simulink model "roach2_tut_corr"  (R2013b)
settings: Solver=VariableStepDiscrete  SolverMode=SingleTasking  StartTime=0.0  StopTime=100  RelTol=1e-3
undefined symbols (not defined in the file): add_latency, addr_width, Bit, bitfield, BitWidth, bram_latency, burst_size, casper_library_scopes, conv_latency, data_width, DelayLen, fan_latency, FFTSize, FFTStage, getfield, increment, led, Location, Lower, mult_latency, mux_latency, n_bits, n_bits_data, n_inputs, n_streams, n_taps, neg_latency, negate_latency, nsamples, pfb_size, pulse_len, reset_period, ROACH, ROACH2, snapshot, sx475t, sync_period, sync_period_bits, Upper, UseCounter, Width
libraries: xbsIndex_r4 x24444, casper_library_misc x73, xbsReplacements_r4 x34, casper_library_delays x14, xps_library x7
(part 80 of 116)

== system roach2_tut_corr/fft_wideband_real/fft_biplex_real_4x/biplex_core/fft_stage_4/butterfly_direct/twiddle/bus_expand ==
  bus_in : Inport
  reinterpret1 : xbsIndex_r4/Reinterpret  force_arith_type=on  arith_type=Unsigned  force_bin_pt=on  bin_pt=0  block_type=reinterpret
  reinterpret2 : xbsIndex_r4/Reinterpret  force_arith_type=on  arith_type=Unsigned  force_bin_pt=on  bin_pt=0  block_type=reinterpret
  slice1 : xbsIndex_r4/Slice  nbits=145  boolean_output=off  mode=Upper Bit Location + Width  bit1=-144  base1=MSB of Input  bit0=0  base0=LSB of Input  dbl_ovrd=off  block_type=slice
  slice2 : xbsIndex_r4/Slice  nbits=144  boolean_output=off  mode=Upper Bit Location + Width  bit1=0  base1=MSB of Input  bit0=0  base0=LSB of Input  dbl_ovrd=off  block_type=slice
  msb_out2 : Outport
  lsb_out1 : Outport  Port=2
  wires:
  bus_in/1 -> slice2/1, slice1/1
  slice2/1 -> reinterpret2/1
  reinterpret2/1 -> msb_out2/1
  slice1/1 -> reinterpret1/1
  reinterpret1/1 -> lsb_out1/1

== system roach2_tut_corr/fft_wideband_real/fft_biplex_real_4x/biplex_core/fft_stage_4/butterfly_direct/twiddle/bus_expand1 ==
  bus_in : Inport
  reinterpret1 : xbsIndex_r4/Reinterpret  force_arith_type=on  arith_type=Unsigned  force_bin_pt=on  bin_pt=0  block_type=reinterpret
  slice1 : xbsIndex_r4/Slice  nbits=144  boolean_output=off  mode=Upper Bit Location + Width  bit1=-1  base1=MSB of Input  bit0=0  base0=LSB of Input  dbl_ovrd=off  block_type=slice
  slice2 : xbsIndex_r4/Slice  nbits=1  boolean_output=on  mode=Upper Bit Location + Width  bit1=0  base1=MSB of Input  bit0=0  base0=LSB of Input  dbl_ovrd=off  block_type=slice
  msb_out2 : Outport
  lsb_out1 : Outport  Port=2
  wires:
  bus_in/1 -> slice2/1, slice1/1
  slice2/1 -> msb_out2/1
  slice1/1 -> reinterpret1/1
  reinterpret1/1 -> lsb_out1/1

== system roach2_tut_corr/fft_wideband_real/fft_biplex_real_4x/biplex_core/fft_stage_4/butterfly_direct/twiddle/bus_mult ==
  a : Inport
  b : Inport  Port=2
  misci : Inport  Port=3
  a*b_bussify : Subsystem  AncestorBlock=casper_library_flow_control/bus_create
  a_debus : Subsystem  AncestorBlock=casper_library_flow_control/bus_expand
  b_debus : Subsystem  AncestorBlock=casper_library_flow_control/bus_expand
  dmisc : xbsIndex_r4/Delay  rst=off  infoeditControl=Selection of Reset will increase slice count due to use of real FFs and instead of SRLs  en=off  latency=mult_latency+add_latency+conv_latency+fan_latency  dbl_ovrd=off  reg_retiming=on  block_type=delay
  mult1 : Subsystem  AncestorBlock=casper_library_multipliers/cmult
  mult2 : Subsystem  AncestorBlock=casper_library_multipliers/cmult
  mult3 : Subsystem  AncestorBlock=casper_library_multipliers/cmult
  mult4 : Subsystem  AncestorBlock=casper_library_multipliers/cmult
  repa : Subsystem  AncestorBlock=casper_library_bus/bus_replicate
  repb : Subsystem  AncestorBlock=casper_library_bus/bus_replicate
  a*b : Outport
  misco : Outport  Port=2
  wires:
  a/1 -> repa/1(in)
  b/1 -> repb/1(in)
  repa/1(out) -> a_debus/1(bus_in)
  repb/1(out) -> b_debus/1(bus_in)
  a_debus/1(msb_lsb_out1) -> mult1/1(a), mult2/1(a), mult3/1(a), mult4/1(a)
  b_debus/1(msb_out4) -> mult1/2(b)
  b_debus/2(out3) -> mult2/2(b)
  b_debus/3(out2) -> mult3/2(b)
  b_debus/4(lsb_out1) -> mult4/2(b)
  misci/1 -> dmisc/1
  mult1/1(ab) -> a*b_bussify/1(in1)
  mult2/1(ab) -> a*b_bussify/2(in2)
  mult3/1(ab) -> a*b_bussify/3(in3)
  mult4/1(ab) -> a*b_bussify/4(in4)
  a*b_bussify/1(bus_out) -> a*b/1
  dmisc/1 -> misco/1

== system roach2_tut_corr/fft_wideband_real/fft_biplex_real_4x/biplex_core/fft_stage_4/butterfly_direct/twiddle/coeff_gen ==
  rst : Inport
  misci : Inport  Port=2
  Counter : xbsIndex_r4/Counter  cnt_type=Free Running  cnt_to=Inf  operation=Up  start_count=0  cnt_by_val=1  arith_type=Unsigned  n_bits=8  bin_pt=0  load_pin=off  rst=on  en=off  explicit_period=on  period=1  dbl_ovrd=off  use_behavioral_HDL=on  implementation=Fabric  block_type=counter
  Slice : xbsIndex_r4/Slice  nbits=3  boolean_output=off  mode=Upper Bit Location + Width  bit1=0  base1=MSB of Input  bit0=0  base0=LSB of Input  dbl_ovrd=off  block_type=slice
  bit_reverse : Subsystem  AncestorBlock=casper_library_misc/bit_reverse
  cosin : Subsystem  Tag=casper:cosin  AncestorBlock=casper_library_downconverter/cosin
  ri_to_c : casper_library_misc/ri_to_c
  w : Outport
  misco : Outport  Port=2
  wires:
  ri_to_c/1 -> w/1
  rst/1 -> Counter/1
  Counter/1 -> Slice/1
  Slice/1 -> bit_reverse/1(in)
  bit_reverse/1(out) -> cosin/1(theta)
  cosin/1(cos) -> ri_to_c/1
  cosin/2(-sin) -> ri_to_c/2
  misci/1 -> cosin/2(misci)
  cosin/3(misco) -> misco/1

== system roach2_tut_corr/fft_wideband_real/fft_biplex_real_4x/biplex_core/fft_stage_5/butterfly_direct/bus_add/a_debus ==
  bus_in : Inport
  reinterpret{1..8} (8 alike) : xbsIndex_r4/Reinterpret  force_arith_type=on  arith_type="Signed  (2's comp)"  force_bin_pt=on  bin_pt=17  block_type=reinterpret
  slice1 : xbsIndex_r4/Slice  nbits=18  boolean_output=off  mode=Upper Bit Location + Width  bit1=-126  base1=MSB of Input  bit0=0  base0=LSB of Input  dbl_ovrd=off  block_type=slice
  slice2 : xbsIndex_r4/Slice  nbits=18  boolean_output=off  mode=Upper Bit Location + Width  bit1=-108  base1=MSB of Input  bit0=0  base0=LSB of Input  dbl_ovrd=off  block_type=slice
  slice3 : xbsIndex_r4/Slice  nbits=18  boolean_output=off  mode=Upper Bit Location + Width  bit1=-90  base1=MSB of Input  bit0=0  base0=LSB of Input  dbl_ovrd=off  block_type=slice
  slice4 : xbsIndex_r4/Slice  nbits=18  boolean_output=off  mode=Upper Bit Location + Width  bit1=-72  base1=MSB of Input  bit0=0  base0=LSB of Input  dbl_ovrd=off  block_type=slice
  slice5 : xbsIndex_r4/Slice  nbits=18  boolean_output=off  mode=Upper Bit Location + Width  bit1=-54  base1=MSB of Input  bit0=0  base0=LSB of Input  dbl_ovrd=off  block_type=slice
  slice6 : xbsIndex_r4/Slice  nbits=18  boolean_output=off  mode=Upper Bit Location + Width  bit1=-36  base1=MSB of Input  bit0=0  base0=LSB of Input  dbl_ovrd=off  block_type=slice
  slice7 : xbsIndex_r4/Slice  nbits=18  boolean_output=off  mode=Upper Bit Location + Width  bit1=-18  base1=MSB of Input  bit0=0  base0=LSB of Input  dbl_ovrd=off  block_type=slice
  slice8 : xbsIndex_r4/Slice  nbits=18  boolean_output=off  mode=Upper Bit Location + Width  bit1=0  base1=MSB of Input  bit0=0  base0=LSB of Input  dbl_ovrd=off  block_type=slice
  msb_out8 : Outport
  out7 : Outport  Port=2
  out6 : Outport  Port=3
  out5 : Outport  Port=4
  out4 : Outport  Port=5
  out3 : Outport  Port=6
  out2 : Outport  Port=7
  lsb_out1 : Outport  Port=8
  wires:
  bus_in/1 -> slice8/1, slice7/1, slice6/1, slice5/1, slice4/1, slice3/1, slice2/1, slice1/1
  slice8/1 -> reinterpret8/1
  reinterpret8/1 -> msb_out8/1
  slice7/1 -> reinterpret7/1
  reinterpret7/1 -> out7/1
  slice6/1 -> reinterpret6/1
  reinterpret6/1 -> out6/1
  slice5/1 -> reinterpret5/1
  reinterpret5/1 -> out5/1
  slice4/1 -> reinterpret4/1
  reinterpret4/1 -> out4/1
  slice3/1 -> reinterpret3/1
  reinterpret3/1 -> out3/1
  slice2/1 -> reinterpret2/1
  reinterpret2/1 -> out2/1
  slice1/1 -> reinterpret1/1
  reinterpret1/1 -> lsb_out1/1

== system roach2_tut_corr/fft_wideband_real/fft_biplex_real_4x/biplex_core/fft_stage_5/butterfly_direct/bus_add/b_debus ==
  bus_in : Inport
  reinterpret{1..8} (8 alike) : xbsIndex_r4/Reinterpret  force_arith_type=on  arith_type="Signed  (2's comp)"  force_bin_pt=on  bin_pt=17  block_type=reinterpret
  slice1 : xbsIndex_r4/Slice  nbits=19  boolean_output=off  mode=Upper Bit Location + Width  bit1=-133  base1=MSB of Input  bit0=0  base0=LSB of Input  dbl_ovrd=off  block_type=slice
  slice2 : xbsIndex_r4/Slice  nbits=19  boolean_output=off  mode=Upper Bit Location + Width  bit1=-114  base1=MSB of Input  bit0=0  base0=LSB of Input  dbl_ovrd=off  block_type=slice
  slice3 : xbsIndex_r4/Slice  nbits=19  boolean_output=off  mode=Upper Bit Location + Width  bit1=-95  base1=MSB of Input  bit0=0  base0=LSB of Input  dbl_ovrd=off  block_type=slice
  slice4 : xbsIndex_r4/Slice  nbits=19  boolean_output=off  mode=Upper Bit Location + Width  bit1=-76  base1=MSB of Input  bit0=0  base0=LSB of Input  dbl_ovrd=off  block_type=slice
  slice5 : xbsIndex_r4/Slice  nbits=19  boolean_output=off  mode=Upper Bit Location + Width  bit1=-57  base1=MSB of Input  bit0=0  base0=LSB of Input  dbl_ovrd=off  block_type=slice
  slice6 : xbsIndex_r4/Slice  nbits=19  boolean_output=off  mode=Upper Bit Location + Width  bit1=-38  base1=MSB of Input  bit0=0  base0=LSB of Input  dbl_ovrd=off  block_type=slice
  slice7 : xbsIndex_r4/Slice  nbits=19  boolean_output=off  mode=Upper Bit Location + Width  bit1=-19  base1=MSB of Input  bit0=0  base0=LSB of Input  dbl_ovrd=off  block_type=slice
  slice8 : xbsIndex_r4/Slice  nbits=19  boolean_output=off  mode=Upper Bit Location + Width  bit1=0  base1=MSB of Input  bit0=0  base0=LSB of Input  dbl_ovrd=off  block_type=slice
  msb_out8 : Outport
  out7 : Outport  Port=2
  out6 : Outport  Port=3
  out5 : Outport  Port=4
  out4 : Outport  Port=5
  out3 : Outport  Port=6
  out2 : Outport  Port=7
  lsb_out1 : Outport  Port=8
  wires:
  bus_in/1 -> slice8/1, slice7/1, slice6/1, slice5/1, slice4/1, slice3/1, slice2/1, slice1/1
  slice8/1 -> reinterpret8/1
  reinterpret8/1 -> msb_out8/1
  slice7/1 -> reinterpret7/1
  reinterpret7/1 -> out7/1
  slice6/1 -> reinterpret6/1
  reinterpret6/1 -> out6/1
  slice5/1 -> reinterpret5/1
  reinterpret5/1 -> out5/1
  slice4/1 -> reinterpret4/1
  reinterpret4/1 -> out4/1
  slice3/1 -> reinterpret3/1
  reinterpret3/1 -> out3/1
  slice2/1 -> reinterpret2/1
  reinterpret2/1 -> out2/1
  slice1/1 -> reinterpret1/1
  reinterpret1/1 -> lsb_out1/1

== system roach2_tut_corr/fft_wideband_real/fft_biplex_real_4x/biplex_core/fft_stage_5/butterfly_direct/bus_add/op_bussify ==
  in1 : Inport
  in2 : Inport  Port=2
  in3 : Inport  Port=3
  in4 : Inport  Port=4
  in5 : Inport  Port=5
  in6 : Inport  Port=6
  in7 : Inport  Port=7
  in8 : Inport  Port=8
  concatenate : xbsIndex_r4/Concat  num_inputs=8  dbl_ovrd=off  block_type=concat
  reinterpret{1..8} (8 alike) : xbsIndex_r4/Reinterpret  force_arith_type=on  arith_type=Unsigned  force_bin_pt=on  bin_pt=0  block_type=reinterpret
  bus_out : Outport
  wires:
  concatenate/1 -> bus_out/1
  in1/1 -> reinterpret1/1
  reinterpret1/1 -> concatenate/1
  in2/1 -> reinterpret2/1
  reinterpret2/1 -> concatenate/2
  in3/1 -> reinterpret3/1
  reinterpret3/1 -> concatenate/3
  in4/1 -> reinterpret4/1
  reinterpret4/1 -> concatenate/4
  in5/1 -> reinterpret5/1
  reinterpret5/1 -> concatenate/5
  in6/1 -> reinterpret6/1
  reinterpret6/1 -> concatenate/6
  in7/1 -> reinterpret7/1
  reinterpret7/1 -> concatenate/7
  in8/1 -> reinterpret8/1
  reinterpret8/1 -> concatenate/8

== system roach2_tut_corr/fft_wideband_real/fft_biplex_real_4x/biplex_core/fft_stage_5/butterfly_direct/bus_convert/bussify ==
  in1 : Inport
  in2 : Inport  Port=2
  in3 : Inport  Port=3
  in4 : Inport  Port=4
  in5 : Inport  Port=5
  in6 : Inport  Port=6
  in7 : Inport  Port=7
  in8 : Inport  Port=8
  in9 : Inport  Port=9
  in10 : Inport  Port=10
  in11 : Inport  Port=11
  in12 : Inport  Port=12
  in13 : Inport  Port=13
  in14 : Inport  Port=14
  in15 : Inport  Port=15
  in16 : Inport  Port=16
  concatenate : xbsIndex_r4/Concat  num_inputs=16  dbl_ovrd=off  block_type=concat
  reinterpret{1..16} (16 alike) : xbsIndex_r4/Reinterpret  force_arith_type=on  arith_type=Unsigned  force_bin_pt=on  bin_pt=0  block_type=reinterpret
  bus_out : Outport
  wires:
  concatenate/1 -> bus_out/1
  in1/1 -> reinterpret1/1
  reinterpret1/1 -> concatenate/1
  in2/1 -> reinterpret2/1
  reinterpret2/1 -> concatenate/2
  in3/1 -> reinterpret3/1
  reinterpret3/1 -> concatenate/3
  in4/1 -> reinterpret4/1
  reinterpret4/1 -> concatenate/4
  in5/1 -> reinterpret5/1
  reinterpret5/1 -> concatenate/5
  in6/1 -> reinterpret6/1
  reinterpret6/1 -> concatenate/6
  in7/1 -> reinterpret7/1
  reinterpret7/1 -> concatenate/7
  in8/1 -> reinterpret8/1
  reinterpret8/1 -> concatenate/8
  in9/1 -> reinterpret9/1
  reinterpret9/1 -> concatenate/9
  in10/1 -> reinterpret10/1
  reinterpret10/1 -> concatenate/10
  in11/1 -> reinterpret11/1
  reinterpret11/1 -> concatenate/11
  in12/1 -> reinterpret12/1
  reinterpret12/1 -> concatenate/12
  in13/1 -> reinterpret13/1
  reinterpret13/1 -> concatenate/13
  in14/1 -> reinterpret14/1
  reinterpret14/1 -> concatenate/14
  in15/1 -> reinterpret15/1
  reinterpret15/1 -> concatenate/15
  in16/1 -> reinterpret16/1
  reinterpret16/1 -> concatenate/16

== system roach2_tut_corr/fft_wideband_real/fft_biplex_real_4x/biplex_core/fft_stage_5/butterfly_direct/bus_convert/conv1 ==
  din : Inport
  all_0s : xbsIndex_r4/Logical  logical_function=NAND  inputs=3  en=off  latency=1  precision=Full  arith_type=Unsigned  n_bits=16  bin_pt=0  align_bp=on  dbl_ovrd=off  block_type=logical
  all_1s : xbsIndex_r4/Logical  logical_function=NAND  inputs=3  en=off  latency=1  precision=Full  arith_type=Unsigned  n_bits=16  bin_pt=0  align_bp=on  dbl_ovrd=off  block_type=logical
  and : xbsIndex_r4/Logical  logical_function=AND  inputs=2  en=off  latency=0  precision=Full  arith_type=Unsigned  n_bits=16  bin_pt=0  align_bp=on  dbl_ovrd=off  block_type=logical
  convert : Subsystem  AncestorBlock=casper_library_misc/convert
  invert1 : xbsIndex_r4/Inverter  en=off  latency=0  dbl_ovrd=off  block_type=inv
  invert2 : xbsIndex_r4/Inverter  en=off  latency=0  dbl_ovrd=off  block_type=inv
  invert3 : xbsIndex_r4/Inverter  en=off  latency=0  dbl_ovrd=off  block_type=inv
  slice1 : xbsIndex_r4/Slice  nbits=1  boolean_output=on  mode=Upper Bit Location + Width  bit1=0  base1=MSB of Input  bit0=0  base0=LSB of Input  dbl_ovrd=off  block_type=slice
  slice2 : xbsIndex_r4/Slice  nbits=1  boolean_output=on  mode=Upper Bit Location + Width  bit1=-1  base1=MSB of Input  bit0=0  base0=LSB of Input  dbl_ovrd=off  block_type=slice
  slice3 : xbsIndex_r4/Slice  nbits=1  boolean_output=on  mode=Upper Bit Location + Width  bit1=-2  base1=MSB of Input  bit0=0  base0=LSB of Input  dbl_ovrd=off  block_type=slice
  dout : Outport
  of : Outport  Port=2
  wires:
  din/1 -> convert/1(in), slice1/1, slice2/1, slice3/1
  convert/1(out) -> dout/1
  slice1/1 -> all_1s/1, invert1/1
  invert1/1 -> all_0s/1
  slice2/1 -> all_1s/2, invert2/1
  invert2/1 -> all_0s/2
  slice3/1 -> all_1s/3, invert3/1
  invert3/1 -> all_0s/3
  all_0s/1 -> and/1
  all_1s/1 -> and/2
  and/1 -> of/1

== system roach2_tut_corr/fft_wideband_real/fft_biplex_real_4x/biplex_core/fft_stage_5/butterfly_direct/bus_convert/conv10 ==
  din : Inport
  all_0s : xbsIndex_r4/Logical  logical_function=NAND  inputs=3  en=off  latency=1  precision=Full  arith_type=Unsigned  n_bits=16  bin_pt=0  align_bp=on  dbl_ovrd=off  block_type=logical
  all_1s : xbsIndex_r4/Logical  logical_function=NAND  inputs=3  en=off  latency=1  precision=Full  arith_type=Unsigned  n_bits=16  bin_pt=0  align_bp=on  dbl_ovrd=off  block_type=logical
  and : xbsIndex_r4/Logical  logical_function=AND  inputs=2  en=off  latency=0  precision=Full  arith_type=Unsigned  n_bits=16  bin_pt=0  align_bp=on  dbl_ovrd=off  block_type=logical
  convert : Subsystem  AncestorBlock=casper_library_misc/convert
  invert1 : xbsIndex_r4/Inverter  en=off  latency=0  dbl_ovrd=off  block_type=inv
  invert2 : xbsIndex_r4/Inverter  en=off  latency=0  dbl_ovrd=off  block_type=inv
  invert3 : xbsIndex_r4/Inverter  en=off  latency=0  dbl_ovrd=off  block_type=inv
  slice1 : xbsIndex_r4/Slice  nbits=1  boolean_output=on  mode=Upper Bit Location + Width  bit1=0  base1=MSB of Input  bit0=0  base0=LSB of Input  dbl_ovrd=off  block_type=slice
  slice2 : xbsIndex_r4/Slice  nbits=1  boolean_output=on  mode=Upper Bit Location + Width  bit1=-1  base1=MSB of Input  bit0=0  base0=LSB of Input  dbl_ovrd=off  block_type=slice
  slice3 : xbsIndex_r4/Slice  nbits=1  boolean_output=on  mode=Upper Bit Location + Width  bit1=-2  base1=MSB of Input  bit0=0  base0=LSB of Input  dbl_ovrd=off  block_type=slice
  dout : Outport
  of : Outport  Port=2
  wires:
  din/1 -> convert/1(in), slice1/1, slice2/1, slice3/1
  convert/1(out) -> dout/1
  slice1/1 -> all_1s/1, invert1/1
  invert1/1 -> all_0s/1
  slice2/1 -> all_1s/2, invert2/1
  invert2/1 -> all_0s/2
  slice3/1 -> all_1s/3, invert3/1
  invert3/1 -> all_0s/3
  all_0s/1 -> and/1
  all_1s/1 -> and/2
  and/1 -> of/1

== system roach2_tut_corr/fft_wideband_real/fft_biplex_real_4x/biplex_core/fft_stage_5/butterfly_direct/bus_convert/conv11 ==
  din : Inport
  all_0s : xbsIndex_r4/Logical  logical_function=NAND  inputs=3  en=off  latency=1  precision=Full  arith_type=Unsigned  n_bits=16  bin_pt=0  align_bp=on  dbl_ovrd=off  block_type=logical
  all_1s : xbsIndex_r4/Logical  logical_function=NAND  inputs=3  en=off  latency=1  precision=Full  arith_type=Unsigned  n_bits=16  bin_pt=0  align_bp=on  dbl_ovrd=off  block_type=logical
  and : xbsIndex_r4/Logical  logical_function=AND  inputs=2  en=off  latency=0  precision=Full  arith_type=Unsigned  n_bits=16  bin_pt=0  align_bp=on  dbl_ovrd=off  block_type=logical
  convert : Subsystem  AncestorBlock=casper_library_misc/convert
  invert1 : xbsIndex_r4/Inverter  en=off  latency=0  dbl_ovrd=off  block_type=inv
  invert2 : xbsIndex_r4/Inverter  en=off  latency=0  dbl_ovrd=off  block_type=inv
  invert3 : xbsIndex_r4/Inverter  en=off  latency=0  dbl_ovrd=off  block_type=inv
  slice1 : xbsIndex_r4/Slice  nbits=1  boolean_output=on  mode=Upper Bit Location + Width  bit1=0  base1=MSB of Input  bit0=0  base0=LSB of Input  dbl_ovrd=off  block_type=slice
  slice2 : xbsIndex_r4/Slice  nbits=1  boolean_output=on  mode=Upper Bit Location + Width  bit1=-1  base1=MSB of Input  bit0=0  base0=LSB of Input  dbl_ovrd=off  block_type=slice
  slice3 : xbsIndex_r4/Slice  nbits=1  boolean_output=on  mode=Upper Bit Location + Width  bit1=-2  base1=MSB of Input  bit0=0  base0=LSB of Input  dbl_ovrd=off  block_type=slice
  dout : Outport
  of : Outport  Port=2
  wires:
  din/1 -> convert/1(in), slice1/1, slice2/1, slice3/1
  convert/1(out) -> dout/1
  slice1/1 -> all_1s/1, invert1/1
  invert1/1 -> all_0s/1
  slice2/1 -> all_1s/2, invert2/1
  invert2/1 -> all_0s/2
  slice3/1 -> all_1s/3, invert3/1
  invert3/1 -> all_0s/3
  all_0s/1 -> and/1
  all_1s/1 -> and/2
  and/1 -> of/1

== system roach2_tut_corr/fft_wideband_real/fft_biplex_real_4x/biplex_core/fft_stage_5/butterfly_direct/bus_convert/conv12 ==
  din : Inport
  all_0s : xbsIndex_r4/Logical  logical_function=NAND  inputs=3  en=off  latency=1  precision=Full  arith_type=Unsigned  n_bits=16  bin_pt=0  align_bp=on  dbl_ovrd=off  block_type=logical
  all_1s : xbsIndex_r4/Logical  logical_function=NAND  inputs=3  en=off  latency=1  precision=Full  arith_type=Unsigned  n_bits=16  bin_pt=0  align_bp=on  dbl_ovrd=off  block_type=logical
  and : xbsIndex_r4/Logical  logical_function=AND  inputs=2  en=off  latency=0  precision=Full  arith_type=Unsigned  n_bits=16  bin_pt=0  align_bp=on  dbl_ovrd=off  block_type=logical
  convert : Subsystem  AncestorBlock=casper_library_misc/convert
  invert1 : xbsIndex_r4/Inverter  en=off  latency=0  dbl_ovrd=off  block_type=inv
  invert2 : xbsIndex_r4/Inverter  en=off  latency=0  dbl_ovrd=off  block_type=inv
  invert3 : xbsIndex_r4/Inverter  en=off  latency=0  dbl_ovrd=off  block_type=inv
  slice1 : xbsIndex_r4/Slice  nbits=1  boolean_output=on  mode=Upper Bit Location + Width  bit1=0  base1=MSB of Input  bit0=0  base0=LSB of Input  dbl_ovrd=off  block_type=slice
  slice2 : xbsIndex_r4/Slice  nbits=1  boolean_output=on  mode=Upper Bit Location + Width  bit1=-1  base1=MSB of Input  bit0=0  base0=LSB of Input  dbl_ovrd=off  block_type=slice
  slice3 : xbsIndex_r4/Slice  nbits=1  boolean_output=on  mode=Upper Bit Location + Width  bit1=-2  base1=MSB of Input  bit0=0  base0=LSB of Input  dbl_ovrd=off  block_type=slice
  dout : Outport
  of : Outport  Port=2
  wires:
  din/1 -> convert/1(in), slice1/1, slice2/1, slice3/1
  convert/1(out) -> dout/1
  slice1/1 -> all_1s/1, invert1/1
  invert1/1 -> all_0s/1
  slice2/1 -> all_1s/2, invert2/1
  invert2/1 -> all_0s/2
  slice3/1 -> all_1s/3, invert3/1
  invert3/1 -> all_0s/3
  all_0s/1 -> and/1
  all_1s/1 -> and/2
  and/1 -> of/1

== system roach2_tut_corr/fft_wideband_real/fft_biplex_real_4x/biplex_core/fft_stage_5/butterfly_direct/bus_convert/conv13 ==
  din : Inport
  all_0s : xbsIndex_r4/Logical  logical_function=NAND  inputs=3  en=off  latency=1  precision=Full  arith_type=Unsigned  n_bits=16  bin_pt=0  align_bp=on  dbl_ovrd=off  block_type=logical
  all_1s : xbsIndex_r4/Logical  logical_function=NAND  inputs=3  en=off  latency=1  precision=Full  arith_type=Unsigned  n_bits=16  bin_pt=0  align_bp=on  dbl_ovrd=off  block_type=logical
  and : xbsIndex_r4/Logical  logical_function=AND  inputs=2  en=off  latency=0  precision=Full  arith_type=Unsigned  n_bits=16  bin_pt=0  align_bp=on  dbl_ovrd=off  block_type=logical
  convert : Subsystem  AncestorBlock=casper_library_misc/convert
  invert1 : xbsIndex_r4/Inverter  en=off  latency=0  dbl_ovrd=off  block_type=inv
  invert2 : xbsIndex_r4/Inverter  en=off  latency=0  dbl_ovrd=off  block_type=inv
  invert3 : xbsIndex_r4/Inverter  en=off  latency=0  dbl_ovrd=off  block_type=inv
  slice1 : xbsIndex_r4/Slice  nbits=1  boolean_output=on  mode=Upper Bit Location + Width  bit1=0  base1=MSB of Input  bit0=0  base0=LSB of Input  dbl_ovrd=off  block_type=slice
  slice2 : xbsIndex_r4/Slice  nbits=1  boolean_output=on  mode=Upper Bit Location + Width  bit1=-1  base1=MSB of Input  bit0=0  base0=LSB of Input  dbl_ovrd=off  block_type=slice
  slice3 : xbsIndex_r4/Slice  nbits=1  boolean_output=on  mode=Upper Bit Location + Width  bit1=-2  base1=MSB of Input  bit0=0  base0=LSB of Input  dbl_ovrd=off  block_type=slice
  dout : Outport
  of : Outport  Port=2
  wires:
  din/1 -> convert/1(in), slice1/1, slice2/1, slice3/1
  convert/1(out) -> dout/1
  slice1/1 -> all_1s/1, invert1/1
  invert1/1 -> all_0s/1
  slice2/1 -> all_1s/2, invert2/1
  invert2/1 -> all_0s/2
  slice3/1 -> all_1s/3, invert3/1
  invert3/1 -> all_0s/3
  all_0s/1 -> and/1
  all_1s/1 -> and/2
  and/1 -> of/1

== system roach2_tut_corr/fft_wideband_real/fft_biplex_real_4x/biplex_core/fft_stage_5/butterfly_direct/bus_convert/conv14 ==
  din : Inport
  all_0s : xbsIndex_r4/Logical  logical_function=NAND  inputs=3  en=off  latency=1  precision=Full  arith_type=Unsigned  n_bits=16  bin_pt=0  align_bp=on  dbl_ovrd=off  block_type=logical
  all_1s : xbsIndex_r4/Logical  logical_function=NAND  inputs=3  en=off  latency=1  precision=Full  arith_type=Unsigned  n_bits=16  bin_pt=0  align_bp=on  dbl_ovrd=off  block_type=logical
  and : xbsIndex_r4/Logical  logical_function=AND  inputs=2  en=off  latency=0  precision=Full  arith_type=Unsigned  n_bits=16  bin_pt=0  align_bp=on  dbl_ovrd=off  block_type=logical
  convert : Subsystem  AncestorBlock=casper_library_misc/convert
  invert1 : xbsIndex_r4/Inverter  en=off  latency=0  dbl_ovrd=off  block_type=inv
  invert2 : xbsIndex_r4/Inverter  en=off  latency=0  dbl_ovrd=off  block_type=inv
  invert3 : xbsIndex_r4/Inverter  en=off  latency=0  dbl_ovrd=off  block_type=inv
  slice1 : xbsIndex_r4/Slice  nbits=1  boolean_output=on  mode=Upper Bit Location + Width  bit1=0  base1=MSB of Input  bit0=0  base0=LSB of Input  dbl_ovrd=off  block_type=slice
  slice2 : xbsIndex_r4/Slice  nbits=1  boolean_output=on  mode=Upper Bit Location + Width  bit1=-1  base1=MSB of Input  bit0=0  base0=LSB of Input  dbl_ovrd=off  block_type=slice
  slice3 : xbsIndex_r4/Slice  nbits=1  boolean_output=on  mode=Upper Bit Location + Width  bit1=-2  base1=MSB of Input  bit0=0  base0=LSB of Input  dbl_ovrd=off  block_type=slice
  dout : Outport
  of : Outport  Port=2
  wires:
  din/1 -> convert/1(in), slice1/1, slice2/1, slice3/1
  convert/1(out) -> dout/1
  slice1/1 -> all_1s/1, invert1/1
  invert1/1 -> all_0s/1
  slice2/1 -> all_1s/2, invert2/1
  invert2/1 -> all_0s/2
  slice3/1 -> all_1s/3, invert3/1
  invert3/1 -> all_0s/3
  all_0s/1 -> and/1
  all_1s/1 -> and/2
  and/1 -> of/1

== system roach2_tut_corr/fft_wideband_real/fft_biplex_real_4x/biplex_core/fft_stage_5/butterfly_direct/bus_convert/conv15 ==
  din : Inport
  all_0s : xbsIndex_r4/Logical  logical_function=NAND  inputs=3  en=off  latency=1  precision=Full  arith_type=Unsigned  n_bits=16  bin_pt=0  align_bp=on  dbl_ovrd=off  block_type=logical
  all_1s : xbsIndex_r4/Logical  logical_function=NAND  inputs=3  en=off  latency=1  precision=Full  arith_type=Unsigned  n_bits=16  bin_pt=0  align_bp=on  dbl_ovrd=off  block_type=logical
  and : xbsIndex_r4/Logical  logical_function=AND  inputs=2  en=off  latency=0  precision=Full  arith_type=Unsigned  n_bits=16  bin_pt=0  align_bp=on  dbl_ovrd=off  block_type=logical
  convert : Subsystem  AncestorBlock=casper_library_misc/convert
  invert1 : xbsIndex_r4/Inverter  en=off  latency=0  dbl_ovrd=off  block_type=inv
  invert2 : xbsIndex_r4/Inverter  en=off  latency=0  dbl_ovrd=off  block_type=inv
  invert3 : xbsIndex_r4/Inverter  en=off  latency=0  dbl_ovrd=off  block_type=inv
  slice1 : xbsIndex_r4/Slice  nbits=1  boolean_output=on  mode=Upper Bit Location + Width  bit1=0  base1=MSB of Input  bit0=0  base0=LSB of Input  dbl_ovrd=off  block_type=slice
  slice2 : xbsIndex_r4/Slice  nbits=1  boolean_output=on  mode=Upper Bit Location + Width  bit1=-1  base1=MSB of Input  bit0=0  base0=LSB of Input  dbl_ovrd=off  block_type=slice
  slice3 : xbsIndex_r4/Slice  nbits=1  boolean_output=on  mode=Upper Bit Location + Width  bit1=-2  base1=MSB of Input  bit0=0  base0=LSB of Input  dbl_ovrd=off  block_type=slice
  dout : Outport
  of : Outport  Port=2
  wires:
  din/1 -> convert/1(in), slice1/1, slice2/1, slice3/1
  convert/1(out) -> dout/1
  slice1/1 -> all_1s/1, invert1/1
  invert1/1 -> all_0s/1
  slice2/1 -> all_1s/2, invert2/1
  invert2/1 -> all_0s/2
  slice3/1 -> all_1s/3, invert3/1
  invert3/1 -> all_0s/3
  all_0s/1 -> and/1
  all_1s/1 -> and/2
  and/1 -> of/1

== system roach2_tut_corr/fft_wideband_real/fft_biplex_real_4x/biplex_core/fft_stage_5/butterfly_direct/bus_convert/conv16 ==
  din : Inport
  all_0s : xbsIndex_r4/Logical  logical_function=NAND  inputs=3  en=off  latency=1  precision=Full  arith_type=Unsigned  n_bits=16  bin_pt=0  align_bp=on  dbl_ovrd=off  block_type=logical
  all_1s : xbsIndex_r4/Logical  logical_function=NAND  inputs=3  en=off  latency=1  precision=Full  arith_type=Unsigned  n_bits=16  bin_pt=0  align_bp=on  dbl_ovrd=off  block_type=logical
  and : xbsIndex_r4/Logical  logical_function=AND  inputs=2  en=off  latency=0  precision=Full  arith_type=Unsigned  n_bits=16  bin_pt=0  align_bp=on  dbl_ovrd=off  block_type=logical
  convert : Subsystem  AncestorBlock=casper_library_misc/convert
  invert1 : xbsIndex_r4/Inverter  en=off  latency=0  dbl_ovrd=off  block_type=inv
  invert2 : xbsIndex_r4/Inverter  en=off  latency=0  dbl_ovrd=off  block_type=inv
  invert3 : xbsIndex_r4/Inverter  en=off  latency=0  dbl_ovrd=off  block_type=inv
  slice1 : xbsIndex_r4/Slice  nbits=1  boolean_output=on  mode=Upper Bit Location + Width  bit1=0  base1=MSB of Input  bit0=0  base0=LSB of Input  dbl_ovrd=off  block_type=slice
  slice2 : xbsIndex_r4/Slice  nbits=1  boolean_output=on  mode=Upper Bit Location + Width  bit1=-1  base1=MSB of Input  bit0=0  base0=LSB of Input  dbl_ovrd=off  block_type=slice
  slice3 : xbsIndex_r4/Slice  nbits=1  boolean_output=on  mode=Upper Bit Location + Width  bit1=-2  base1=MSB of Input  bit0=0  base0=LSB of Input  dbl_ovrd=off  block_type=slice
  dout : Outport
  of : Outport  Port=2
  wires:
  din/1 -> convert/1(in), slice1/1, slice2/1, slice3/1
  convert/1(out) -> dout/1
  slice1/1 -> all_1s/1, invert1/1
  invert1/1 -> all_0s/1
  slice2/1 -> all_1s/2, invert2/1
  invert2/1 -> all_0s/2
  slice3/1 -> all_1s/3, invert3/1
  invert3/1 -> all_0s/3
  all_0s/1 -> and/1
  all_1s/1 -> and/2
  and/1 -> of/1

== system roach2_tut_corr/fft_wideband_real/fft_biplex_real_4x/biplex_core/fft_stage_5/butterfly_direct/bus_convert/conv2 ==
  din : Inport
  all_0s : xbsIndex_r4/Logical  logical_function=NAND  inputs=3  en=off  latency=1  precision=Full  arith_type=Unsigned  n_bits=16  bin_pt=0  align_bp=on  dbl_ovrd=off  block_type=logical
  all_1s : xbsIndex_r4/Logical  logical_function=NAND  inputs=3  en=off  latency=1  precision=Full  arith_type=Unsigned  n_bits=16  bin_pt=0  align_bp=on  dbl_ovrd=off  block_type=logical
  and : xbsIndex_r4/Logical  logical_function=AND  inputs=2  en=off  latency=0  precision=Full  arith_type=Unsigned  n_bits=16  bin_pt=0  align_bp=on  dbl_ovrd=off  block_type=logical
  convert : Subsystem  AncestorBlock=casper_library_misc/convert
  invert1 : xbsIndex_r4/Inverter  en=off  latency=0  dbl_ovrd=off  block_type=inv
  invert2 : xbsIndex_r4/Inverter  en=off  latency=0  dbl_ovrd=off  block_type=inv
  invert3 : xbsIndex_r4/Inverter  en=off  latency=0  dbl_ovrd=off  block_type=inv
  slice1 : xbsIndex_r4/Slice  nbits=1  boolean_output=on  mode=Upper Bit Location + Width  bit1=0  base1=MSB of Input  bit0=0  base0=LSB of Input  dbl_ovrd=off  block_type=slice
  slice2 : xbsIndex_r4/Slice  nbits=1  boolean_output=on  mode=Upper Bit Location + Width  bit1=-1  base1=MSB of Input  bit0=0  base0=LSB of Input  dbl_ovrd=off  block_type=slice
  slice3 : xbsIndex_r4/Slice  nbits=1  boolean_output=on  mode=Upper Bit Location + Width  bit1=-2  base1=MSB of Input  bit0=0  base0=LSB of Input  dbl_ovrd=off  block_type=slice
  dout : Outport
  of : Outport  Port=2
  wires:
  din/1 -> convert/1(in), slice1/1, slice2/1, slice3/1
  convert/1(out) -> dout/1
  slice1/1 -> all_1s/1, invert1/1
  invert1/1 -> all_0s/1
  slice2/1 -> all_1s/2, invert2/1
  invert2/1 -> all_0s/2
  slice3/1 -> all_1s/3, invert3/1
  invert3/1 -> all_0s/3
  all_0s/1 -> and/1
  all_1s/1 -> and/2
  and/1 -> of/1

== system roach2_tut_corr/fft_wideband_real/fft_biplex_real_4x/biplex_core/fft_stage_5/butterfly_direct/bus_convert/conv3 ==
  din : Inport
  all_0s : xbsIndex_r4/Logical  logical_function=NAND  inputs=3  en=off  latency=1  precision=Full  arith_type=Unsigned  n_bits=16  bin_pt=0  align_bp=on  dbl_ovrd=off  block_type=logical
  all_1s : xbsIndex_r4/Logical  logical_function=NAND  inputs=3  en=off  latency=1  precision=Full  arith_type=Unsigned  n_bits=16  bin_pt=0  align_bp=on  dbl_ovrd=off  block_type=logical
  and : xbsIndex_r4/Logical  logical_function=AND  inputs=2  en=off  latency=0  precision=Full  arith_type=Unsigned  n_bits=16  bin_pt=0  align_bp=on  dbl_ovrd=off  block_type=logical
  convert : Subsystem  AncestorBlock=casper_library_misc/convert
  invert1 : xbsIndex_r4/Inverter  en=off  latency=0  dbl_ovrd=off  block_type=inv
  invert2 : xbsIndex_r4/Inverter  en=off  latency=0  dbl_ovrd=off  block_type=inv
  invert3 : xbsIndex_r4/Inverter  en=off  latency=0  dbl_ovrd=off  block_type=inv
  slice1 : xbsIndex_r4/Slice  nbits=1  boolean_output=on  mode=Upper Bit Location + Width  bit1=0  base1=MSB of Input  bit0=0  base0=LSB of Input  dbl_ovrd=off  block_type=slice
  slice2 : xbsIndex_r4/Slice  nbits=1  boolean_output=on  mode=Upper Bit Location + Width  bit1=-1  base1=MSB of Input  bit0=0  base0=LSB of Input  dbl_ovrd=off  block_type=slice
  slice3 : xbsIndex_r4/Slice  nbits=1  boolean_output=on  mode=Upper Bit Location + Width  bit1=-2  base1=MSB of Input  bit0=0  base0=LSB of Input  dbl_ovrd=off  block_type=slice
  dout : Outport
  of : Outport  Port=2
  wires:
  din/1 -> convert/1(in), slice1/1, slice2/1, slice3/1
  convert/1(out) -> dout/1
  slice1/1 -> all_1s/1, invert1/1
  invert1/1 -> all_0s/1
  slice2/1 -> all_1s/2, invert2/1
  invert2/1 -> all_0s/2
  slice3/1 -> all_1s/3, invert3/1
  invert3/1 -> all_0s/3
  all_0s/1 -> and/1
  all_1s/1 -> and/2
  and/1 -> of/1

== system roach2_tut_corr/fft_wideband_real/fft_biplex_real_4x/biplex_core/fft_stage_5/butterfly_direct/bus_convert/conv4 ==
  din : Inport
  all_0s : xbsIndex_r4/Logical  logical_function=NAND  inputs=3  en=off  latency=1  precision=Full  arith_type=Unsigned  n_bits=16  bin_pt=0  align_bp=on  dbl_ovrd=off  block_type=logical
  all_1s : xbsIndex_r4/Logical  logical_function=NAND  inputs=3  en=off  latency=1  precision=Full  arith_type=Unsigned  n_bits=16  bin_pt=0  align_bp=on  dbl_ovrd=off  block_type=logical
  and : xbsIndex_r4/Logical  logical_function=AND  inputs=2  en=off  latency=0  precision=Full  arith_type=Unsigned  n_bits=16  bin_pt=0  align_bp=on  dbl_ovrd=off  block_type=logical
  convert : Subsystem  AncestorBlock=casper_library_misc/convert
  invert1 : xbsIndex_r4/Inverter  en=off  latency=0  dbl_ovrd=off  block_type=inv
  invert2 : xbsIndex_r4/Inverter  en=off  latency=0  dbl_ovrd=off  block_type=inv
  invert3 : xbsIndex_r4/Inverter  en=off  latency=0  dbl_ovrd=off  block_type=inv
  slice1 : xbsIndex_r4/Slice  nbits=1  boolean_output=on  mode=Upper Bit Location + Width  bit1=0  base1=MSB of Input  bit0=0  base0=LSB of Input  dbl_ovrd=off  block_type=slice
  slice2 : xbsIndex_r4/Slice  nbits=1  boolean_output=on  mode=Upper Bit Location + Width  bit1=-1  base1=MSB of Input  bit0=0  base0=LSB of Input  dbl_ovrd=off  block_type=slice
  slice3 : xbsIndex_r4/Slice  nbits=1  boolean_output=on  mode=Upper Bit Location + Width  bit1=-2  base1=MSB of Input  bit0=0  base0=LSB of Input  dbl_ovrd=off  block_type=slice
  dout : Outport
  of : Outport  Port=2
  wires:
  din/1 -> convert/1(in), slice1/1, slice2/1, slice3/1
  convert/1(out) -> dout/1
  slice1/1 -> all_1s/1, invert1/1
  invert1/1 -> all_0s/1
  slice2/1 -> all_1s/2, invert2/1
  invert2/1 -> all_0s/2
  slice3/1 -> all_1s/3, invert3/1
  invert3/1 -> all_0s/3
  all_0s/1 -> and/1
  all_1s/1 -> and/2
  and/1 -> of/1

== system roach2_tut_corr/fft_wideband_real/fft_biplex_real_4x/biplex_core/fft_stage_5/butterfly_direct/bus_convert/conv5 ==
  din : Inport
  all_0s : xbsIndex_r4/Logical  logical_function=NAND  inputs=3  en=off  latency=1  precision=Full  arith_type=Unsigned  n_bits=16  bin_pt=0  align_bp=on  dbl_ovrd=off  block_type=logical
  all_1s : xbsIndex_r4/Logical  logical_function=NAND  inputs=3  en=off  latency=1  precision=Full  arith_type=Unsigned  n_bits=16  bin_pt=0  align_bp=on  dbl_ovrd=off  block_type=logical
  and : xbsIndex_r4/Logical  logical_function=AND  inputs=2  en=off  latency=0  precision=Full  arith_type=Unsigned  n_bits=16  bin_pt=0  align_bp=on  dbl_ovrd=off  block_type=logical
  convert : Subsystem  AncestorBlock=casper_library_misc/convert
  invert1 : xbsIndex_r4/Inverter  en=off  latency=0  dbl_ovrd=off  block_type=inv
  invert2 : xbsIndex_r4/Inverter  en=off  latency=0  dbl_ovrd=off  block_type=inv
  invert3 : xbsIndex_r4/Inverter  en=off  latency=0  dbl_ovrd=off  block_type=inv
  slice1 : xbsIndex_r4/Slice  nbits=1  boolean_output=on  mode=Upper Bit Location + Width  bit1=0  base1=MSB of Input  bit0=0  base0=LSB of Input  dbl_ovrd=off  block_type=slice
  slice2 : xbsIndex_r4/Slice  nbits=1  boolean_output=on  mode=Upper Bit Location + Width  bit1=-1  base1=MSB of Input  bit0=0  base0=LSB of Input  dbl_ovrd=off  block_type=slice
  slice3 : xbsIndex_r4/Slice  nbits=1  boolean_output=on  mode=Upper Bit Location + Width  bit1=-2  base1=MSB of Input  bit0=0  base0=LSB of Input  dbl_ovrd=off  block_type=slice
  dout : Outport
  of : Outport  Port=2
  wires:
  din/1 -> convert/1(in), slice1/1, slice2/1, slice3/1
  convert/1(out) -> dout/1
  slice1/1 -> all_1s/1, invert1/1
  invert1/1 -> all_0s/1
  slice2/1 -> all_1s/2, invert2/1
  invert2/1 -> all_0s/2
  slice3/1 -> all_1s/3, invert3/1
  invert3/1 -> all_0s/3
  all_0s/1 -> and/1
  all_1s/1 -> and/2
  and/1 -> of/1

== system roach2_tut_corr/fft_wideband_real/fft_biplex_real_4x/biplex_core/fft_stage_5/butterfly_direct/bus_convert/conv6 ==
  din : Inport
  all_0s : xbsIndex_r4/Logical  logical_function=NAND  inputs=3  en=off  latency=1  precision=Full  arith_type=Unsigned  n_bits=16  bin_pt=0  align_bp=on  dbl_ovrd=off  block_type=logical
  all_1s : xbsIndex_r4/Logical  logical_function=NAND  inputs=3  en=off  latency=1  precision=Full  arith_type=Unsigned  n_bits=16  bin_pt=0  align_bp=on  dbl_ovrd=off  block_type=logical
  and : xbsIndex_r4/Logical  logical_function=AND  inputs=2  en=off  latency=0  precision=Full  arith_type=Unsigned  n_bits=16  bin_pt=0  align_bp=on  dbl_ovrd=off  block_type=logical
  convert : Subsystem  AncestorBlock=casper_library_misc/convert
  invert1 : xbsIndex_r4/Inverter  en=off  latency=0  dbl_ovrd=off  block_type=inv
  invert2 : xbsIndex_r4/Inverter  en=off  latency=0  dbl_ovrd=off  block_type=inv
  invert3 : xbsIndex_r4/Inverter  en=off  latency=0  dbl_ovrd=off  block_type=inv
  slice1 : xbsIndex_r4/Slice  nbits=1  boolean_output=on  mode=Upper Bit Location + Width  bit1=0  base1=MSB of Input  bit0=0  base0=LSB of Input  dbl_ovrd=off  block_type=slice
  slice2 : xbsIndex_r4/Slice  nbits=1  boolean_output=on  mode=Upper Bit Location + Width  bit1=-1  base1=MSB of Input  bit0=0  base0=LSB of Input  dbl_ovrd=off  block_type=slice
  slice3 : xbsIndex_r4/Slice  nbits=1  boolean_output=on  mode=Upper Bit Location + Width  bit1=-2  base1=MSB of Input  bit0=0  base0=LSB of Input  dbl_ovrd=off  block_type=slice
  dout : Outport
  of : Outport  Port=2
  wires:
  din/1 -> convert/1(in), slice1/1, slice2/1, slice3/1
  convert/1(out) -> dout/1
  slice1/1 -> all_1s/1, invert1/1
  invert1/1 -> all_0s/1
  slice2/1 -> all_1s/2, invert2/1
  invert2/1 -> all_0s/2
  slice3/1 -> all_1s/3, invert3/1
  invert3/1 -> all_0s/3
  all_0s/1 -> and/1
  all_1s/1 -> and/2
  and/1 -> of/1

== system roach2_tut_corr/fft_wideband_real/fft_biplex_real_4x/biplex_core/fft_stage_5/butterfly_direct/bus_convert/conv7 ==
  din : Inport
  all_0s : xbsIndex_r4/Logical  logical_function=NAND  inputs=3  en=off  latency=1  precision=Full  arith_type=Unsigned  n_bits=16  bin_pt=0  align_bp=on  dbl_ovrd=off  block_type=logical
  all_1s : xbsIndex_r4/Logical  logical_function=NAND  inputs=3  en=off  latency=1  precision=Full  arith_type=Unsigned  n_bits=16  bin_pt=0  align_bp=on  dbl_ovrd=off  block_type=logical
  and : xbsIndex_r4/Logical  logical_function=AND  inputs=2  en=off  latency=0  precision=Full  arith_type=Unsigned  n_bits=16  bin_pt=0  align_bp=on  dbl_ovrd=off  block_type=logical
  convert : Subsystem  AncestorBlock=casper_library_misc/convert
  invert1 : xbsIndex_r4/Inverter  en=off  latency=0  dbl_ovrd=off  block_type=inv
  invert2 : xbsIndex_r4/Inverter  en=off  latency=0  dbl_ovrd=off  block_type=inv
  invert3 : xbsIndex_r4/Inverter  en=off  latency=0  dbl_ovrd=off  block_type=inv
  slice1 : xbsIndex_r4/Slice  nbits=1  boolean_output=on  mode=Upper Bit Location + Width  bit1=0  base1=MSB of Input  bit0=0  base0=LSB of Input  dbl_ovrd=off  block_type=slice
  slice2 : xbsIndex_r4/Slice  nbits=1  boolean_output=on  mode=Upper Bit Location + Width  bit1=-1  base1=MSB of Input  bit0=0  base0=LSB of Input  dbl_ovrd=off  block_type=slice
  slice3 : xbsIndex_r4/Slice  nbits=1  boolean_output=on  mode=Upper Bit Location + Width  bit1=-2  base1=MSB of Input  bit0=0  base0=LSB of Input  dbl_ovrd=off  block_type=slice
  dout : Outport
  of : Outport  Port=2
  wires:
  din/1 -> convert/1(in), slice1/1, slice2/1, slice3/1
  convert/1(out) -> dout/1
  slice1/1 -> all_1s/1, invert1/1
  invert1/1 -> all_0s/1
  slice2/1 -> all_1s/2, invert2/1
  invert2/1 -> all_0s/2
  slice3/1 -> all_1s/3, invert3/1
  invert3/1 -> all_0s/3
  all_0s/1 -> and/1
  all_1s/1 -> and/2
  and/1 -> of/1

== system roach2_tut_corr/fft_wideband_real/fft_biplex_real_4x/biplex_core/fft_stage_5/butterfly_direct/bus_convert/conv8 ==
  din : Inport
  all_0s : xbsIndex_r4/Logical  logical_function=NAND  inputs=3  en=off  latency=1  precision=Full  arith_type=Unsigned  n_bits=16  bin_pt=0  align_bp=on  dbl_ovrd=off  block_type=logical
  all_1s : xbsIndex_r4/Logical  logical_function=NAND  inputs=3  en=off  latency=1  precision=Full  arith_type=Unsigned  n_bits=16  bin_pt=0  align_bp=on  dbl_ovrd=off  block_type=logical
  and : xbsIndex_r4/Logical  logical_function=AND  inputs=2  en=off  latency=0  precision=Full  arith_type=Unsigned  n_bits=16  bin_pt=0  align_bp=on  dbl_ovrd=off  block_type=logical
  convert : Subsystem  AncestorBlock=casper_library_misc/convert
  invert1 : xbsIndex_r4/Inverter  en=off  latency=0  dbl_ovrd=off  block_type=inv
  invert2 : xbsIndex_r4/Inverter  en=off  latency=0  dbl_ovrd=off  block_type=inv
  invert3 : xbsIndex_r4/Inverter  en=off  latency=0  dbl_ovrd=off  block_type=inv
  slice1 : xbsIndex_r4/Slice  nbits=1  boolean_output=on  mode=Upper Bit Location + Width  bit1=0  base1=MSB of Input  bit0=0  base0=LSB of Input  dbl_ovrd=off  block_type=slice
  slice2 : xbsIndex_r4/Slice  nbits=1  boolean_output=on  mode=Upper Bit Location + Width  bit1=-1  base1=MSB of Input  bit0=0  base0=LSB of Input  dbl_ovrd=off  block_type=slice
  slice3 : xbsIndex_r4/Slice  nbits=1  boolean_output=on  mode=Upper Bit Location + Width  bit1=-2  base1=MSB of Input  bit0=0  base0=LSB of Input  dbl_ovrd=off  block_type=slice
  dout : Outport
  of : Outport  Port=2
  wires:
  din/1 -> convert/1(in), slice1/1, slice2/1, slice3/1
  convert/1(out) -> dout/1
  slice1/1 -> all_1s/1, invert1/1
  invert1/1 -> all_0s/1
  slice2/1 -> all_1s/2, invert2/1
  invert2/1 -> all_0s/2
  slice3/1 -> all_1s/3, invert3/1
  invert3/1 -> all_0s/3
  all_0s/1 -> and/1
  all_1s/1 -> and/2
  and/1 -> of/1

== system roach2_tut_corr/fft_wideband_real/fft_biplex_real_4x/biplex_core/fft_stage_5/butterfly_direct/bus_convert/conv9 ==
  din : Inport
  all_0s : xbsIndex_r4/Logical  logical_function=NAND  inputs=3  en=off  latency=1  precision=Full  arith_type=Unsigned  n_bits=16  bin_pt=0  align_bp=on  dbl_ovrd=off  block_type=logical
  all_1s : xbsIndex_r4/Logical  logical_function=NAND  inputs=3  en=off  latency=1  precision=Full  arith_type=Unsigned  n_bits=16  bin_pt=0  align_bp=on  dbl_ovrd=off  block_type=logical
  and : xbsIndex_r4/Logical  logical_function=AND  inputs=2  en=off  latency=0  precision=Full  arith_type=Unsigned  n_bits=16  bin_pt=0  align_bp=on  dbl_ovrd=off  block_type=logical
  convert : Subsystem  AncestorBlock=casper_library_misc/convert
  invert1 : xbsIndex_r4/Inverter  en=off  latency=0  dbl_ovrd=off  block_type=inv
  invert2 : xbsIndex_r4/Inverter  en=off  latency=0  dbl_ovrd=off  block_type=inv
  invert3 : xbsIndex_r4/Inverter  en=off  latency=0  dbl_ovrd=off  block_type=inv
  slice1 : xbsIndex_r4/Slice  nbits=1  boolean_output=on  mode=Upper Bit Location + Width  bit1=0  base1=MSB of Input  bit0=0  base0=LSB of Input  dbl_ovrd=off  block_type=slice
  slice2 : xbsIndex_r4/Slice  nbits=1  boolean_output=on  mode=Upper Bit Location + Width  bit1=-1  base1=MSB of Input  bit0=0  base0=LSB of Input  dbl_ovrd=off  block_type=slice
  slice3 : xbsIndex_r4/Slice  nbits=1  boolean_output=on  mode=Upper Bit Location + Width  bit1=-2  base1=MSB of Input  bit0=0  base0=LSB of Input  dbl_ovrd=off  block_type=slice
  dout : Outport
  of : Outport  Port=2
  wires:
  din/1 -> convert/1(in), slice1/1, slice2/1, slice3/1
  convert/1(out) -> dout/1
  slice1/1 -> all_1s/1, invert1/1
  invert1/1 -> all_0s/1
  slice2/1 -> all_1s/2, invert2/1
  invert2/1 -> all_0s/2
  slice3/1 -> all_1s/3, invert3/1
  invert3/1 -> all_0s/3
  all_0s/1 -> and/1
  all_1s/1 -> and/2
  and/1 -> of/1

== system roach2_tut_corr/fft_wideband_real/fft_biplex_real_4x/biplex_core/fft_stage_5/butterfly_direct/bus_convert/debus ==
  bus_in : Inport
  reinterpret{1..16} (16 alike) : xbsIndex_r4/Reinterpret  force_arith_type=on  arith_type="Signed  (2's comp)"  force_bin_pt=on  bin_pt=18  block_type=reinterpret
  slice1 : xbsIndex_r4/Slice  nbits=21  boolean_output=off  mode=Upper Bit Location + Width  bit1=-315  base1=MSB of Input  bit0=0  base0=LSB of Input  dbl_ovrd=off  block_type=slice
  slice10 : xbsIndex_r4/Slice  nbits=21  boolean_output=off  mode=Upper Bit Location + Width  bit1=-126  base1=MSB of Input  bit0=0  base0=LSB of Input  dbl_ovrd=off  block_type=slice
  slice11 : xbsIndex_r4/Slice  nbits=21  boolean_output=off  mode=Upper Bit Location + Width  bit1=-105  base1=MSB of Input  bit0=0  base0=LSB of Input  dbl_ovrd=off  block_type=slice
  slice12 : xbsIndex_r4/Slice  nbits=21  boolean_output=off  mode=Upper Bit Location + Width  bit1=-84  base1=MSB of Input  bit0=0  base0=LSB of Input  dbl_ovrd=off  block_type=slice
  slice13 : xbsIndex_r4/Slice  nbits=21  boolean_output=off  mode=Upper Bit Location + Width  bit1=-63  base1=MSB of Input  bit0=0  base0=LSB of Input  dbl_ovrd=off  block_type=slice
  slice14 : xbsIndex_r4/Slice  nbits=21  boolean_output=off  mode=Upper Bit Location + Width  bit1=-42  base1=MSB of Input  bit0=0  base0=LSB of Input  dbl_ovrd=off  block_type=slice
  slice15 : xbsIndex_r4/Slice  nbits=21  boolean_output=off  mode=Upper Bit Location + Width  bit1=-21  base1=MSB of Input  bit0=0  base0=LSB of Input  dbl_ovrd=off  block_type=slice
  slice16 : xbsIndex_r4/Slice  nbits=21  boolean_output=off  mode=Upper Bit Location + Width  bit1=0  base1=MSB of Input  bit0=0  base0=LSB of Input  dbl_ovrd=off  block_type=slice
  slice2 : xbsIndex_r4/Slice  nbits=21  boolean_output=off  mode=Upper Bit Location + Width  bit1=-294  base1=MSB of Input  bit0=0  base0=LSB of Input  dbl_ovrd=off  block_type=slice
  slice3 : xbsIndex_r4/Slice  nbits=21  boolean_output=off  mode=Upper Bit Location + Width  bit1=-273  base1=MSB of Input  bit0=0  base0=LSB of Input  dbl_ovrd=off  block_type=slice
  slice4 : xbsIndex_r4/Slice  nbits=21  boolean_output=off  mode=Upper Bit Location + Width  bit1=-252  base1=MSB of Input  bit0=0  base0=LSB of Input  dbl_ovrd=off  block_type=slice
  slice5 : xbsIndex_r4/Slice  nbits=21  boolean_output=off  mode=Upper Bit Location + Width  bit1=-231  base1=MSB of Input  bit0=0  base0=LSB of Input  dbl_ovrd=off  block_type=slice
  slice6 : xbsIndex_r4/Slice  nbits=21  boolean_output=off  mode=Upper Bit Location + Width  bit1=-210  base1=MSB of Input  bit0=0  base0=LSB of Input  dbl_ovrd=off  block_type=slice
  slice7 : xbsIndex_r4/Slice  nbits=21  boolean_output=off  mode=Upper Bit Location + Width  bit1=-189  base1=MSB of Input  bit0=0  base0=LSB of Input  dbl_ovrd=off  block_type=slice
  slice8 : xbsIndex_r4/Slice  nbits=21  boolean_output=off  mode=Upper Bit Location + Width  bit1=-168  base1=MSB of Input  bit0=0  base0=LSB of Input  dbl_ovrd=off  block_type=slice
  slice9 : xbsIndex_r4/Slice  nbits=21  boolean_output=off  mode=Upper Bit Location + Width  bit1=-147  base1=MSB of Input  bit0=0  base0=LSB of Input  dbl_ovrd=off  block_type=slice
  msb_out16 : Outport
  out15 : Outport  Port=2
  out14 : Outport  Port=3
  out13 : Outport  Port=4
  out12 : Outport  Port=5
  out11 : Outport  Port=6
  out10 : Outport  Port=7
  out9 : Outport  Port=8
  out8 : Outport  Port=9
  out7 : Outport  Port=10
  out6 : Outport  Port=11
  out5 : Outport  Port=12
  out4 : Outport  Port=13
  out3 : Outport  Port=14
  out2 : Outport  Port=15
  lsb_out1 : Outport  Port=16
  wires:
  bus_in/1 -> slice16/1, slice15/1, slice14/1, slice13/1, slice12/1, slice11/1, slice10/1, slice9/1, slice8/1, slice7/1, slice6/1, slice5/1, slice4/1, slice3/1, slice2/1, slice1/1
  slice16/1 -> reinterpret16/1
  reinterpret16/1 -> msb_out16/1
  slice15/1 -> reinterpret15/1
  reinterpret15/1 -> out15/1
  slice14/1 -> reinterpret14/1
  reinterpret14/1 -> out14/1
  slice13/1 -> reinterpret13/1
  reinterpret13/1 -> out13/1
  slice12/1 -> reinterpret12/1
  reinterpret12/1 -> out12/1
  slice11/1 -> reinterpret11/1
  reinterpret11/1 -> out11/1
  slice10/1 -> reinterpret10/1
  reinterpret10/1 -> out10/1
  slice9/1 -> reinterpret9/1
  reinterpret9/1 -> out9/1
  slice8/1 -> reinterpret8/1
  reinterpret8/1 -> out8/1
  slice7/1 -> reinterpret7/1
  reinterpret7/1 -> out7/1
  slice6/1 -> reinterpret6/1
  reinterpret6/1 -> out6/1
  slice5/1 -> reinterpret5/1
  reinterpret5/1 -> out5/1
  slice4/1 -> reinterpret4/1
  reinterpret4/1 -> out4/1
  slice3/1 -> reinterpret3/1
  reinterpret3/1 -> out3/1
  slice2/1 -> reinterpret2/1
  reinterpret2/1 -> out2/1
  slice1/1 -> reinterpret1/1
  reinterpret1/1 -> lsb_out1/1
